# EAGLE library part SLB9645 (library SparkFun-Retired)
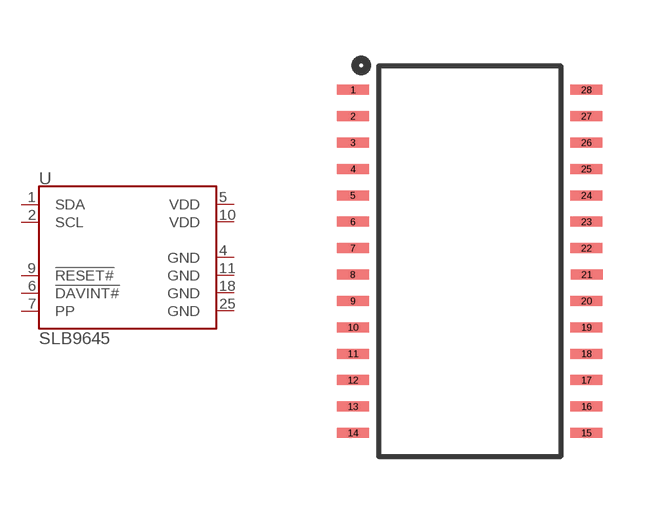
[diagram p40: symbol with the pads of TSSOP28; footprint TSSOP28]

Designator prefix -

## SLB9645 (PROD_ID: IC-XXXX)  [TSSOP28]
1  SDA
2  SCL
4  GND
5  VDD
6  !DAVINT#
7  PP
9  !RESET#
10  VDD
11  GND
18  GND
25  GND

## Footprint TSSOP28 (pad centres in mm)
smd 0.8 x 0.25: 1 -2.921,4.623; 2 -2.921,3.962; 3 -2.921,3.302; 4 -2.921,2.642; 5 -2.921,1.981; 6 -2.921,1.321; 7 -2.921,0.66; 8 -2.927,0; 9 -2.921,-0.66; 10 -2.921,-1.321; 11 -2.921,-1.981; 12 -2.921,-2.642; 13 -2.921,-3.302; 14 -2.921,-3.962; 15 2.921,-3.962; 16 2.921,-3.302; 17 2.921,-2.642; 18 2.921,-1.981; 19 2.921,-1.321; 20 2.921,-0.66; 21 2.927,0; 22 2.921,0.66; 23 2.921,1.321; 24 2.921,1.981; 25 2.921,2.642; 26 2.921,3.302; 27 2.921,3.962; 28 2.921,4.623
